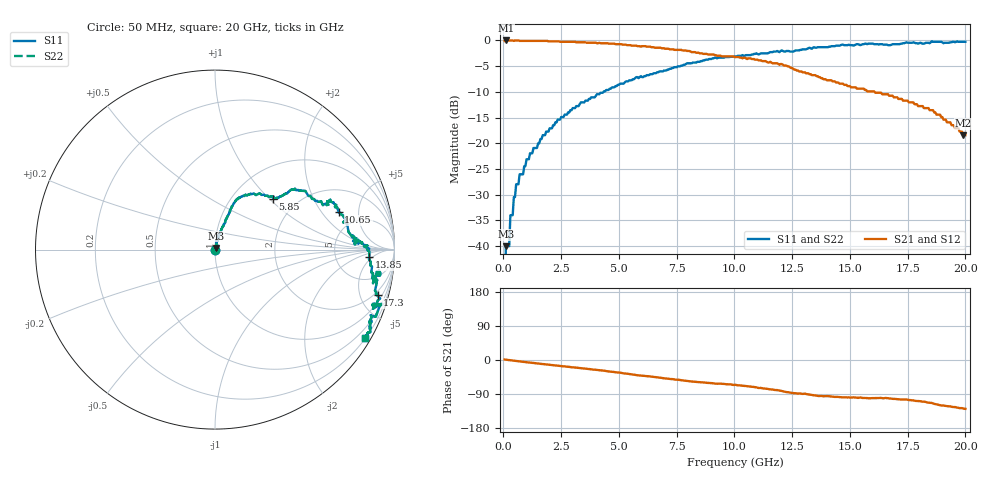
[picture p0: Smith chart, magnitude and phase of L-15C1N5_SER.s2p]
# MHZ S MA R 50
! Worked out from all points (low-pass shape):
!   400 points, 50 MHz to 20 GHz, reference 50 ohm
!   highest |S21| = 0.00 dB at 100 MHz (marker M1); lowest = -18.4 dB at 19.9 GHz (marker M2)
!   |S21| within 3 dB of the highest: start of sweep to 9.41 GHz
!   lowest |S11| = -40.0 dB at 100 MHz (marker M3), VSWR 1.02, Z = 50.5 + j0.881 ohm
!   |S11| at or under -10 dB: start of sweep to 4.331 GHz
!   |S22| runs from - to -0.2 dB; largest |S21 - S12| = 0
!   S11 on the Smith chart (normalised r, x): 50 MHz: 1.00, +0.00; 5.85 GHz: 1.52, +1.05; 10.65 GHz: 3.43, +2.98; 13.85 GHz: 12, -4; 17.3 GHz: 1.60, -6.94; 20 GHz: 0.22, -3.66
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50  0 44.1  0.99 1.4  0.99 1.4  0 44.1
100  0.01 60.7  1 0.9  1 0.9  0.01 60.7
250  0.01 68.3  1 -0.2  1 -0.2  0.01 68.3
300  0.02 73.3  1 -0.6  1 -0.6  0.02 73.3
400  0.02 72.7  1 -1.4  1 -1.4  0.02 72.7
450  0.03 67.2  0.99 -1.7  0.99 -1.7  0.03 67.2
550  0.04 80.6  1 -2.6  1 -2.6  0.04 80.6
1000  0.07 75.2  0.99 -5.8  0.99 -5.8  0.07 75.2
3400  0.25 68.6  0.96 -21.9  0.96 -21.9  0.25 68.6
5850  0.43 41.2  0.88 -40.6  0.88 -40.6  0.43 41.2
6700  0.49 38.5  0.85 -46.3  0.85 -46.3  0.49 38.5
10050  0.7 23.0  0.69 -65.4  0.69 -65.4  0.7 23.0
10650  0.72 16.9  0.67 -69.7  0.67 -69.7  0.72 16.9
11550  0.77 4.9  0.62 -77.6  0.62 -77.6  0.77 4.9
13350  0.83 1.2  0.46 -92.3  0.46 -92.3  0.83 1.2
13850  0.86 -2.8  0.42 -95.6  0.42 -95.6  0.86 -2.8
15050  0.9 -12.0  0.35 -99.2  0.35 -99.2  0.9 -12.0
16700  0.9 -10.1  0.29 -101.4  0.29 -101.4  0.9 -10.1
17300  0.94 -15.6  0.26 -104.4  0.26 -104.4  0.94 -15.6
18600  0.97 -18.9  0.21 -114.7  0.21 -114.7  0.97 -18.9
19900  0.97 -29.5  0.12 -127.8  0.12 -127.8  0.97 -29.5
20000  0.97 -30.5  0.12 -128.9  0.12 -128.9  0.97 -30.5
